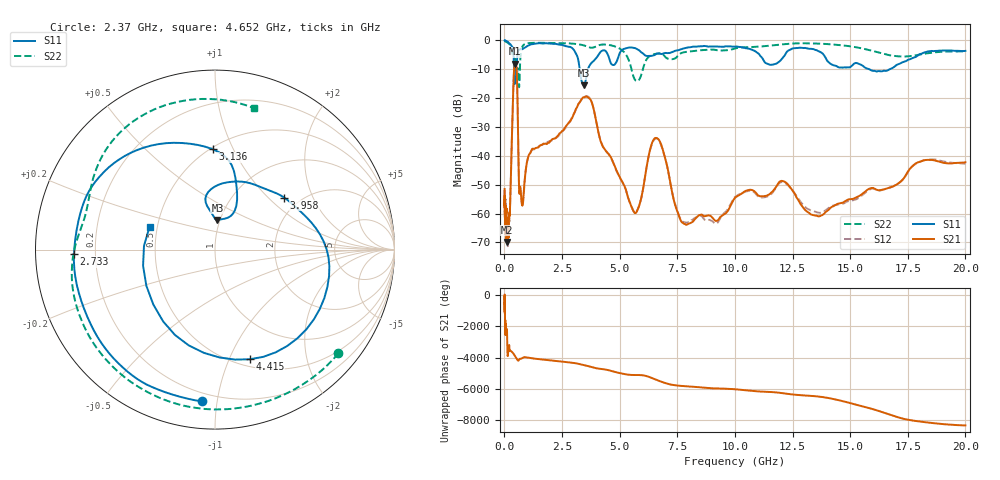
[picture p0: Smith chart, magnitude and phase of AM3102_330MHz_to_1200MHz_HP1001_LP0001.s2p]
! Date/Time: Tue, Sep 11, 2018 5:17 PM
! Network Analyzer: Agilent Technologies E8362B Rev: A.07.50.63
! Sweep from 0.010 to 20.000 GHz, 1601 Points, Sweep Type: LOG
! Power Supply: 4.949 V, 0.001 A
# Hz S DB R 50
!freq MagS11 AngS11 MagS21 AngS21 MagS12 AngS12 MagS22 AngS22
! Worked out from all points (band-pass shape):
!   1601 points, 10 MHz to 20 GHz, reference 50 ohm
!   highest |S21| = -8.05 dB at 458 MHz (marker M1); lowest = -69.8 dB at 96.87 MHz (marker M2)
!   |S21| within 3 dB of the highest: 414 MHz to 536.7 MHz (122.7 MHz wide, 25.8 % of centre)
!   lowest |S11| = -15.6 dB at 3.449 GHz (marker M3), VSWR 1.40, Z = 48.6 + j16.5 ohm
!   |S11| at or under -10 dB: 418.9 MHz to 467 MHz (48.11 MHz wide, 10.9 % of centre); 3.267 GHz to 3.626 GHz (359.1 MHz wide, 10.4 % of centre); 15.84 GHz to 16.71 GHz (870.4 MHz wide, 5.35 % of centre)
!   |S22| runs from -16.2 to -0.2 dB; largest |S21 - S12| = 0.0046
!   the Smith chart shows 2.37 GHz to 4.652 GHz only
!   S11 on the Smith chart (normalised r, x): 2.37 GHz: 0.15, -0.91; 2.733 GHz: 0.12, -0.02; 3.136 GHz: 0.51, +0.84; 3.958 GHz: 1.66, +1.26; 4.415 GHz: 0.58, -1.19; 4.652 GHz: 0.45, +0.14
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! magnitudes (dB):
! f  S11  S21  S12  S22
! 10 MHz  0.0  -51.5  -54.1  -0.2
! 35.55 MHz  0.0  -65.4  -65.4  -0.3
! 96.87 MHz  -0.2  -69.8  -65.2  -0.6
! 126.4 MHz  -0.4  -65.2  -62.9  -0.7
! 234.4 MHz  -1.1  -59.9  -59.8  -1.4
! 447.2 MHz  -14.9  -8.2  -8.2  -6.3
! 458 MHz  -12.5  -8.0  -8.1  -6.4
! 535.7 MHz  -7.7  -10.9  -10.9  -12.1
! 638.6 MHz  -3.2  -51.7  -51.5  -16.2
! 765 MHz  -2.9  -57.0  -56.9  -2.4
! 1.59 GHz  -1.0  -36.3  -36.2  -0.8
! 2.37 GHz  -1.4  -32.4  -32.9  -0.9
! 2.733 GHz  -2.1  -29.1  -29.5  -1.0
! 3.136 GHz  -5.0  -23.4  -23.4  -1.2
! 3.449 GHz  -15.6  -19.7  -19.7  -1.7
! 3.958 GHz  -6.3  -27.1  -27.0  -2.1
! 4.415 GHz  -3.9  -38.4  -38.4  -1.4
! 4.652 GHz  -8.3  -41.0  -41.1  -1.7
! 5.652 GHz  -2.6  -59.8  -59.7  -13.5
! 6.58 GHz  -4.7  -33.8  -34.0  -4.6
! 7.92 GHz  -2.5  -63.9  -63.1  -3.9
! 20 GHz  -3.6  -42.2  -42.7  -3.8
